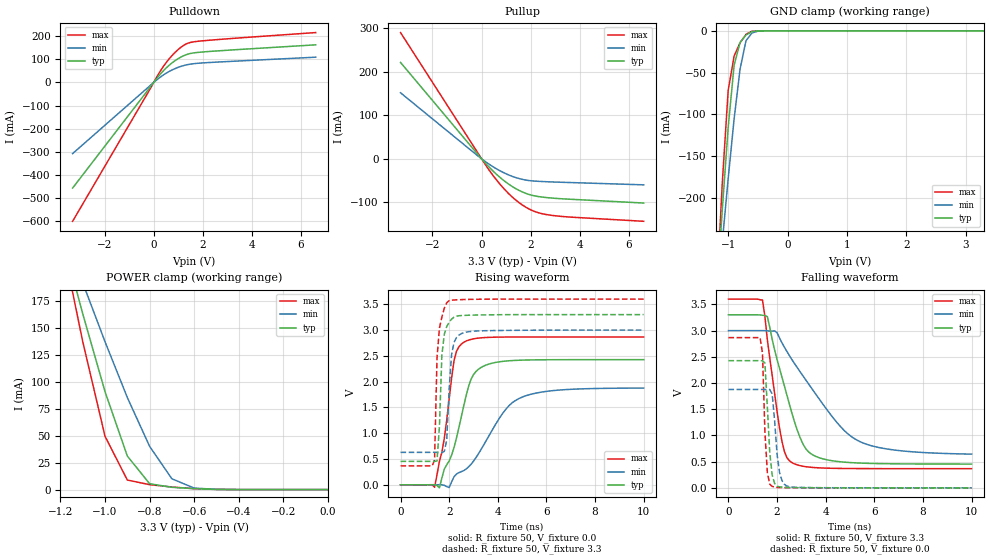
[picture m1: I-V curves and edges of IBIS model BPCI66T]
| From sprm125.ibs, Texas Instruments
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| Reserved Pins
|V6   Reserved
|AA3   Reserved
|AD3   Reserved
|AC4   Reserved
|E14   Reserved
|AF3   Reserved
|AB3   Reserved
|C1   Reserved
|C7   Reserved
|D7   Reserved
|A7   Reserved
|D8   Reserved
|C8   Reserved
|B8   Reserved
|D9   Reserved
|C9   Reserved
|B9   Reserved
|A9   Reserved
|D10   Reserved
|C10   Reserved
|B10   Reserved
|A10   Reserved
|D11   Reserved
|E11   Reserved
|C11   Reserved
|B11   Reserved
|A11   Reserved
|E12   Reserved
|D12   Reserved
|C12   Reserved
|B12   Reserved
|E13   Reserved
|A13   Reserved
|Y26   Reserved
|Y25   Reserved
|W23   Reserved
|Y24   Reserved
|Y23   Reserved
|AA26   Reserved
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[Model]   BPCI66T
|  PCI I/O circuit
Model_type   I/O
Vinh = 2.00
Vinl = 0.80
Enable   Active-Low
Polarity   Non-Inverting
| signals   A, GZ, Y
Vmeas = 1.5
|   typ   min   max
C_comp   1.6056p   1.5280p   1.7919p
|   typ   min   max
[Temperature Range]   25   -40   125
|   typ   min   max
[Voltage Range]   3.30V   3.00V   3.60V
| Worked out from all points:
|   slope of the pulldown table from 0 to 0.495 V, typ, clamps not added: 8.09 ohm
|   slope of the pullup table from 0 to 0.495 V, typ, clamps not added: 16.7 ohm
|   GND clamp passes 1 mA (typ) near -0.60 V on its own axis
|   POWER clamp passes 1 mA (typ) near -0.61 V on its own axis
|   rising waveform, R_fixture 50, V_fixture 0.0: 20-80 % time 801ps typ, 1.54ns min, 499ps max; typ from 0 V to 2.43 V
|   falling waveform, R_fixture 50, V_fixture 3.3: 20-80 % time 1.04ns typ, 2.22ns min, 580ps max; typ from 3.3 V to 0.454 V
|   rising waveform, R_fixture 50, V_fixture 3.3: 20-80 % time 169ps typ, 176ps min, 158ps max; typ from 0.454 V to 3.3 V
|   falling waveform, R_fixture 50, V_fixture 0.0: 20-80 % time 190ps typ, 221ps min, 145ps max; typ from 2.43 V to 0 V
[Pulldown]
|   Voltage   I(typ)   I(min)   I(max)
-3.3V     -456.7mA   -307.6mA   -600.5mA
200mV     27.24mA    17.45mA    37.15mA
600mV     71.61mA    45.73mA    98.17mA
800mV     88.96mA    56.65mA    122.4mA
1.1V      109.4mA    69.26mA    151.5mA
1.4V      122.9mA    77.62mA    170.2mA
1.8V      130.1mA    83.05mA    178.2mA
6.6V      162.9mA    109.5mA    215.9mA
[GND_clamp]
|   Voltage   I(typ)   I(min)   I(max)
-3.3V     -2.845A    -2.152A    -3.683A
-1.2V     -324mA     -334.2mA   -324mA
-1.1V     -215.5mA   -254.2mA   -183.6mA
-1V       -115.9mA   -177.2mA   -71.55mA
-900mV    -41.27mA   -105.6mA   -30.15mA
-800mV    -13.94mA   -45.85mA   -14.45mA
-700mV    -4.994mA   -11.86mA   -4.208mA
-600mV    -963.1uA   -2.542mA   -476.5uA
-500mV    -87.74uA   -433.1uA   -22.26uA
-400mV    -4.9uA     -52.73uA   -497.2nA
3.3V      88.82pA    3.015uA    133.2pA
[Pullup]
|   Voltage   I(typ)   I(min)   I(max)
-3.3V     221.4mA    151.7mA    290mA
-200mV    13.27mA    8.886mA    17.7mA
300mV     -18.67mA   -12.2mA    -25.34mA
600mV     -35.26mA   -22.85mA   -48.04mA
900mV     -49.69mA   -31.89mA   -68.04mA
1.2V      -61.91mA   -39.28mA   -85.27mA
1.5V      -71.82mA   -44.94mA   -99.66mA
1.8V      -79.36mA   -48.82mA   -111.1mA
2.1V      -84.46mA   -50.93mA   -119.6mA
2.7V      -89.38mA   -52.78mA   -128.7mA
3.6V      -92.89mA   -54.52mA   -133.9mA
6.6V      -101.6mA   -59.83mA   -143.6mA
[POWER_clamp]
|   Voltage   I(typ)   I(min)   I(max)
-3.3V     1.995A     1.512A     2.581A
-1.2V     240mA      248.2mA    238mA
-1.1V     163.1mA    191.8mA    137.2mA
-1V       90.81mA    137.1mA    49.45mA
-900mV    31.15mA    85.45mA    8.887mA
-800mV    5.452mA    40.11mA    4.585mA
-700mV    2.137mA    10.02mA    2.412mA
-600mV    899.5uA    1.417mA    878.2uA
-500mV    220.1uA    238.5uA    140uA
0V        577.3pA    14.74nA    133.2pA
[Ramp]
|   I(typ)   I(min)   I(max)
dV/dt_r   1.456/0.795n   1.125/1.538n   1.720/0.490n
dV/dt_f   1.708/1.044n   1.414/2.221n   1.940/0.579n
[Rising Waveform]
R_fixture = 50
V_fixture = 0.0
|  pu_on
|  TIME   V(typ)   V(min)   V(max)
0s        1nV        9nV        1nV
1.4ns     1.925mV    252uV      -48.96mV
1.6ns     -59.82mV   1.139mV    453.5mV
1.8ns     303.6mV    -10.45mV   898.6mV
2.2ns     722.9mV    156mV      2.406V
2.6ns     1.531V     275mV      2.763V
2.9ns     2.046V     397.6mV    2.819V
3.2ns     2.238V     597mV      2.844V
4.9ns     2.415V     1.679V     2.866V
10ns      2.426V     1.875V     2.866V
[Falling Waveform]
R_fixture = 50
V_fixture = 3.3
V_fixture_min = 3.0
V_fixture_max = 3.6
|  pd_on
|  TIME   V(typ)   V(min)   V(max)
0s        3.3V       3V         3.6V
1.4ns     3.292V     3V         3.583V
1.6ns     3.266V     2.996V     2.829V
2.1ns     2.281V     2.86V      1.143V
2.3ns     1.945V     2.684V     696.9mV
2.6ns     1.443V     2.454V     484.9mV
3ns       900.5mV    2.179V     418.1mV
3.4ns     648.9mV    1.913V     392.3mV
5.3ns     475.2mV    908.4mV    368mV
10ns      454mV      645.3mV    366.5mV
[Rising Waveform]
R_fixture = 50
V_fixture = 3.3
V_fixture_min = 3.0
V_fixture_max = 3.6
|  pd_off
|  TIME   V(typ)   V(min)   V(max)
0s        453.7mV    628.5mV    366.5mV
1.4ns     453.6mV    628.5mV    479.5mV
1.5ns     460.1mV    627.9mV    2.455V
1.6ns     1.125V     626.8mV    3.04V
1.7ns     2.51V      625.5mV    3.252V
1.9ns     3.067V     864.9mV    3.53V
2ns       3.152V     1.851V     3.57V
2.2ns     3.249V     2.759V     3.583V
2.6ns     3.284V     2.949V     3.592V
10ns      3.3V       3V         3.6V
[Falling Waveform]
R_fixture = 50
V_fixture = 0.0
|  pu_off
|  TIME   V(typ)   V(min)   V(max)
0s        2.426V     1.877V     2.866V
1.3ns     2.425V     1.877V     2.866V
1.4ns     2.425V     1.877V     2.572V
1.5ns     2.38V      1.876V     1.066V
1.6ns     1.543V     1.877V     292.7mV
1.7ns     664.2mV    1.875V     69.51mV
1.8ns     241.9mV    1.789V     26.97mV
2.1ns     18.83mV    298.4mV    6.33mV
2.4ns     8.259mV    34.74mV    3.533mV
10ns      5.209uV    122.5uV    141nV
